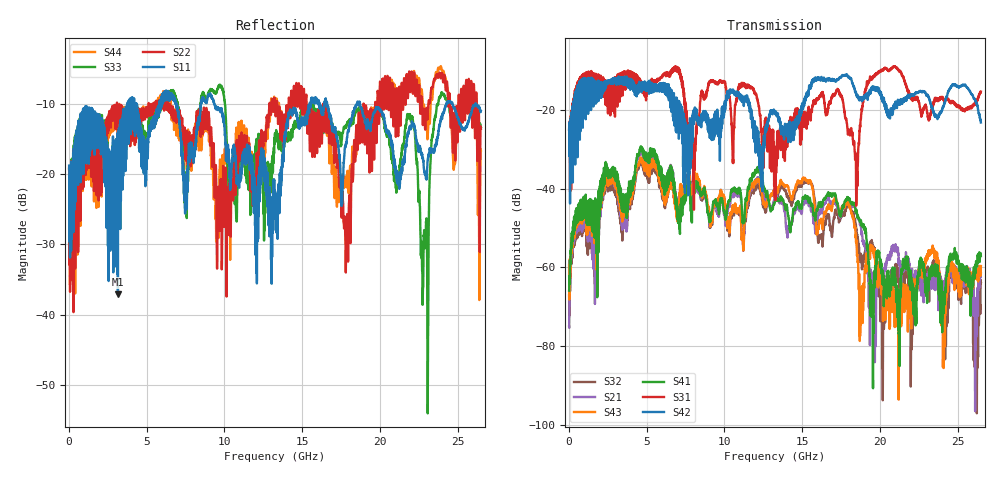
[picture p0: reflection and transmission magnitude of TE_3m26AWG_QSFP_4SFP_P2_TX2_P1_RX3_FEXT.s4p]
!Agilent Technologies,N5222A,MY51421691,A.10.00.00
!Agilent N5222A: A.10.00.00
!Date: Friday, January 30, 2015 12:36:58
!Correction: S11(Full 4 Port(1,2,3,4))
!S12(Full 4 Port(1,2,3,4))
!S13(Full 4 Port(1,2,3,4))
!S14(Full 4 Port(1,2,3,4))
!S21(Full 4 Port(1,2,3,4))
!S22(Full 4 Port(1,2,3,4))
!S23(Full 4 Port(1,2,3,4))
!S24(Full 4 Port(1,2,3,4))
!S31(Full 4 Port(1,2,3,4))
!S32(Full 4 Port(1,2,3,4))
!S33(Full 4 Port(1,2,3,4))
!S34(Full 4 Port(1,2,3,4))
!S41(Full 4 Port(1,2,3,4))
!S42(Full 4 Port(1,2,3,4))
!S43(Full 4 Port(1,2,3,4))
!S44(Full 4 Port(1,2,3,4))
!S4P File: Measurements: <S11,S12,S13,S14>,
!<S21,S22,S23,S24>,
!<S31,S32,S33,S34>,
!<S41,S42,S43,S44>:
# Hz S  dB  R 50.0
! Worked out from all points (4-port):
!   2650 points, 10 MHz to 26.5 GHz, reference 50 ohm
!   strongest paths, dB at 10 MHz, 6.63 GHz, 13.26 GHz, 19.88 GHz, 26.5 GHz:
!     S42: -25.0, -15.9, -20.2, -14.2, -23.1
!     S31: -24.9, -10.2, -30.2, -10.6, -15.3
!     S41: -65.9, -37.3, -43.3, -55.7, -57.1
!     S43: -59.4, -39.7, -40.5, -63.1, -59.7
!     S21: -75.0, -37.1, -42.4, -60.6, -61.5
!     S32: -67.1, -39.9, -40.6, -64.9, -64.0
!   lowest |S11| = -37.1 dB at 3.15 GHz (marker M1), VSWR 1.03, Z = 50.6 - j1.27 ohm
!   |S11| at or under -10 dB: start of sweep to 3.77 GHz; 9.35 GHz to 15.5 GHz (6.146 GHz wide, 49.5 % of centre); 18.72 GHz to 24.29 GHz (5.568 GHz wide, 25.9 % of centre)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
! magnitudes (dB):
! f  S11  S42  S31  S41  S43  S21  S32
! 10 MHz  -18.8  -25.0  -24.9  -65.9  -59.4  -75.0  -67.1
! 3.15 GHz  -37.1  -13.1  -16.9  -37.0  -39.6  -39.2  -41.7
! 12.36 GHz  -21.4  -33.0  -25.4  -37.5  -40.2  -39.6  -41.2
! 17.96 GHz  -13.8  -11.7  -25.7  -42.6  -43.8  -42.4  -43.8
! 18.8 GHz  -10.7  -17.0  -21.0  -48.4  -69.9  -50.2  -58.7
! 19.49 GHz  -12.3  -14.6  -11.9  -68.4  -54.5  -61.8  -53.9
! 26.5 GHz  -11.1  -23.1  -15.3  -57.1  -59.7  -61.5  -64.0
